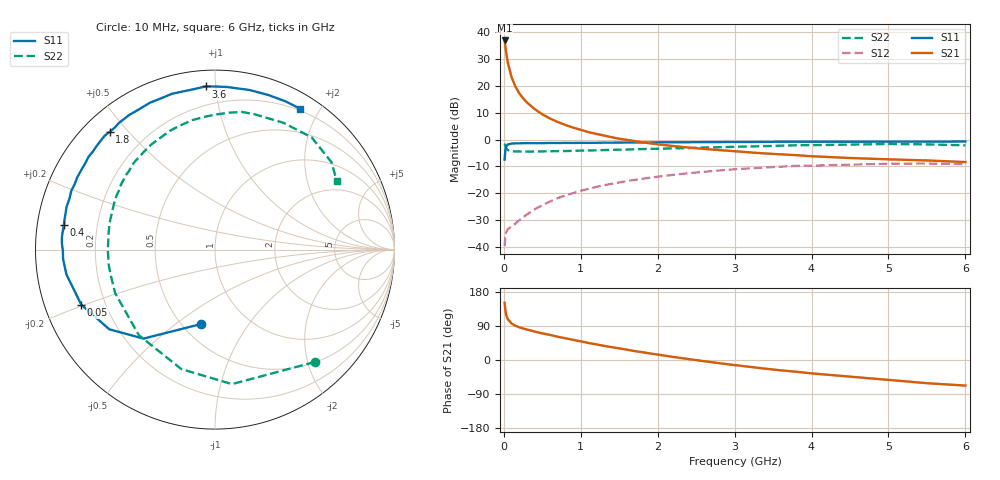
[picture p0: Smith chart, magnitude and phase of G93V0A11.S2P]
! SIEMENS Small Signal Semiconductors
! BFG235
! Si NPN RF Bipolar Junction Transistor in SOT223
! VCE = 3 V  IC = 110 mA
! Common Emitter S-Parameters:  July  1994
# GHz  S  MA  R  50
!  f  S11  S21  S12  S22
! GHz  MAG  ANG  MAG  ANG  MAG  ANG  MAG  ANG
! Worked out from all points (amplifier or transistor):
!   40 points, 10 MHz to 6 GHz, reference 50 ohm
!   highest |S21| = 36.9 dB at 10 MHz (marker M1)
!   |S21| within 3 dB of that: start of sweep to 23.35 MHz
!   unconditionally stable (mu >= 1): 460.6 MHz to 1.53 GHz
!   at 200 MHz: K = 0.79, MSG = 23.7 dB, |S12| = -30.1 dB
!   at 1.5 GHz: K = 1.00, MAG = 7.8 dB, |S12| = -16.0 dB
!   at 6 GHz: K = 0.91, MSG = 0.4 dB, |S12| = -9.2 dB
!   S11 on the Smith chart (normalised r, x): 10 MHz: 0.61, -0.62; 50 MHz: 0.11, -0.20; 400 MHz: 0.08, +0.08; 1.8 GHz: 0.08, +0.45; 3.6 GHz: 0.09, +0.94; 6 GHz: 0.18, +1.76
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0.01  0.4227 -100.8  70 151.1  0.0103 62.3  0.8374 -48.4
0.02  0.6364 -128.8  53.95 131.8  0.0159 46.8  0.7552 -82.8
0.03  0.7376 -143.0  41.88 120.1  0.0186 38.7  0.6918 -105.7
0.05  0.8058 -157.6  27.61 108.0  0.0211 32.6  0.6382 -131.7
0.1  0.8393 -170.5  14.5 96.3  0.0241 34.7  0.6068 -156.4
0.15  0.848 -176.4  9.735 90.4  0.0272 40.9  0.5982 -166.6
0.2  0.8478 -179.6  7.28 86.5  0.0314 45.7  0.5984 -172.4
0.25  0.854 177.5  5.868 83.1  0.0358 49.5  0.596 -176.5
0.3  0.8557 175.3  4.899 80.4  0.0401 51.9  0.5972 -179.9
0.4  0.8535 170.9  3.69 75.0  0.05 55.1  0.5966 175.2
0.5  0.8559 167.2  2.946 70.3  0.0598 56.7  0.6001 171.0
0.7  0.8592 160.6  2.123 61.4  0.0808 56.3  0.6072 163.7
0.9  0.8624 155.2  1.669 53.2  0.1004 53.6  0.6144 157.5
1.1  0.8672 148.8  1.373 44.9  0.1206 50.5  0.6253 151.4
1.4  0.8725 141.4  1.104 33.9  0.1492 44.7  0.6408 142.9
1.8  0.8805 131.7  0.887 20.6  0.1856 36.1  0.6639 131.9
2.2  0.8895 122.7  0.756 8.1  0.2191 27.1  0.6851 121.1
3.2  0.8992 101.3  0.575 -18.2  0.2905 3.9  0.7409 95.1
3.6  0.9106 93.3  0.529 -27.3  0.3119 -6.0  0.7668 84.1
4.5  0.9098 77.8  0.452 -43.9  0.3395 -25.6  0.8028 61.6
5.5  0.9147 64.6  0.407 -61.2  0.357 -47.2  0.8113 36.8
6  0.9169 58.9  0.38 -67.5  0.3471 -55.4  0.7787 29.6
